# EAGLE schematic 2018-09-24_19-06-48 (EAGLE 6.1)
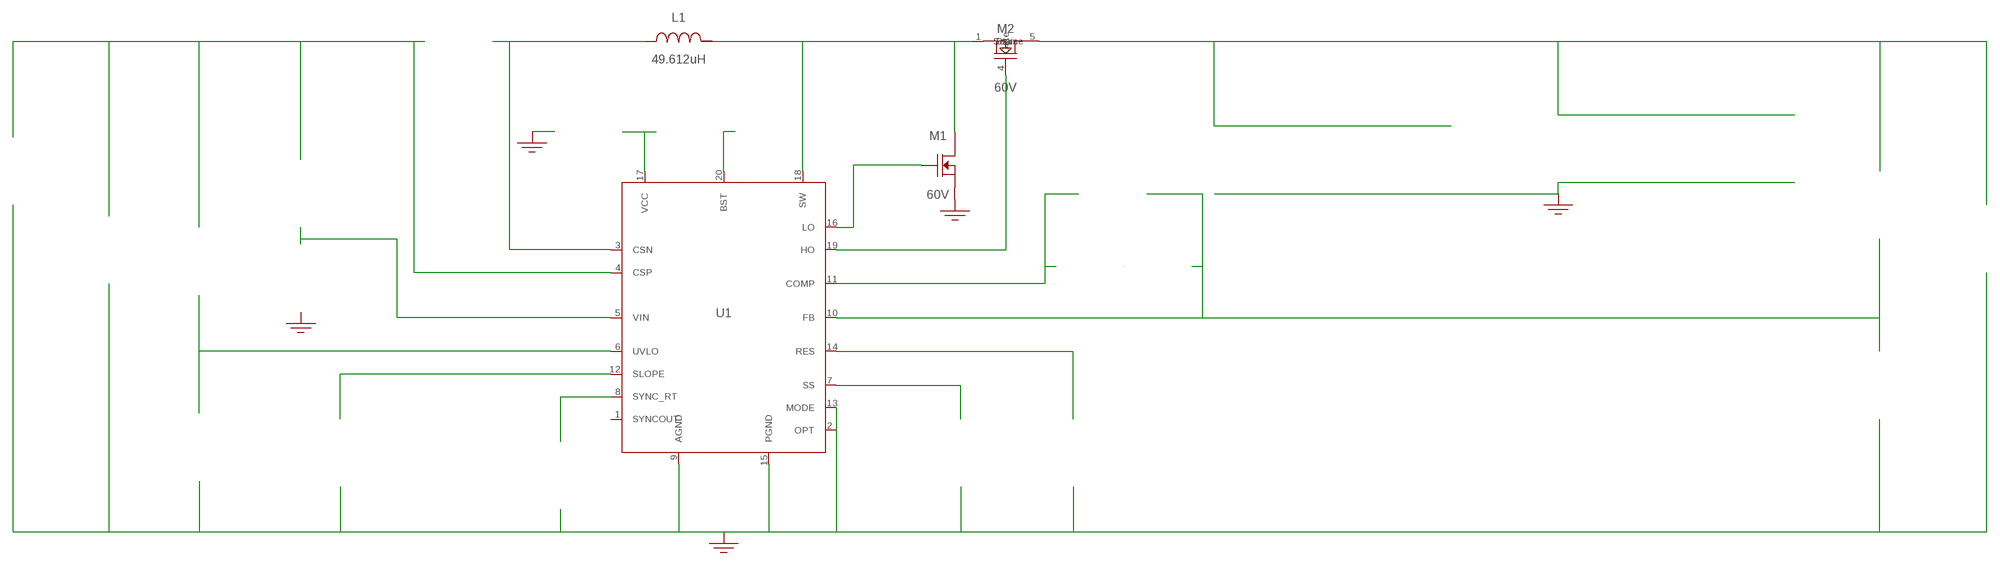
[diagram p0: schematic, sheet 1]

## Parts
CBST  330nF  C1608X5R1H334K080ABC1608X5R1H334K080AB  [0603]  (not placed on a sheet)
CCOMP  27nF  C1812C273J5GACTUC1812C273J5GACTU  [1812]  (not placed on a sheet)
CCOMP2  1.5nF  GCM1885C1H152JA16DGCM1885C1H152JA16D  [0603]  (not placed on a sheet)
CIN  270uF  16SVPG270M16SVPG270M  [CAPSMT_62_C10]  (not placed on a sheet)
COUT  470uF  EEV-FK1J471MEEV-FK1J471M  [SM_RADIAL_J16]  (not placed on a sheet)
COUT_2  470uF  EEV-FK1J471MEEV-FK1J471M  [SM_RADIAL_J16]  (not placed on a sheet)
COUT_3  470uF  EEV-FK1J471MEEV-FK1J471M  [SM_RADIAL_J16]  (not placed on a sheet)
COUT_4  470uF  EEV-FK1J471MEEV-FK1J471M  [SM_RADIAL_J16]  (not placed on a sheet)
COUTX  10uF  CL32B106KBJNNWECL32B106KBJNNWE  [1210_270]  (not placed on a sheet)
COUTX_2  10uF  CL32B106KBJNNWECL32B106KBJNNWE  [1210_270]  (not placed on a sheet)
COUTX_3  10uF  CL32B106KBJNNWECL32B106KBJNNWE  [1210_270]  (not placed on a sheet)
COUTX_4  10uF  CL32B106KBJNNWECL32B106KBJNNWE  [1210_270]  (not placed on a sheet)
CRES  470nF  GRM188R71E474KA12DGRM188R71E474KA12D  [0603]  (not placed on a sheet)
CSS  220nF  GRM155R61A224KE19DGRM155R61A224KE19D  [0402]  (not placed on a sheet)
CVCC  4.7uF  C1608X6S1C475K080ACC1608X6S1C475K080AC  [0603]  (not placed on a sheet)
CVIN  470nF  GRM188R61C474KA93DGRM188R61C474KA93D  [0603]  (not placed on a sheet)
DBST  540mV  XBS104S13R-GXBS104S13R-G  [SOD-323]  (not placed on a sheet)
GND1  WB_GND  WB_GNDWB_GND  [WB_GND]
GND2  WB_GND  WB_GNDWB_GND  [WB_GND]
GND3  WB_GND  WB_GNDWB_GND  [WB_GND]
GND4  WB_GND  WB_GNDWB_GND  [WB_GND]
GND5  WB_GND  WB_GNDWB_GND  [WB_GND]
IOUT  WB_CURRENT_LOAD  WB_CURRENT_LOADWB_CURRENT_LOAD  [WB_CURRENT_LOAD]  (not placed on a sheet)
L1  49.612uH  CUSTOM1CUSTOM1  [GEN_Ind]
M1  60V  CSD18532Q5BCSD18532Q5B  [TRANS_NexFET_Q5B]
M2  60V  CSD18543Q3ACSD18543Q3A  [DNH0008A]
RCOMP  36.5k  RC0201FR-0736K5LRC0201FR-0736K5L  [0201]  (not placed on a sheet)
RFBB  1.6k  RC0603FR-071K6LRC0603FR-071K6L  [0603]  (not placed on a sheet)
RFBT  46.4k  CRCW040246K4FKEDCRCW040246K4FKED  [0402]  (not placed on a sheet)
RSENSE  4m  ERJ-M1WSF4M0UERJ-M1WSF4M0U  [2512]  (not placed on a sheet)
RSLOPE  301k  CRCW0402301KFKEDCRCW0402301KFKED  [0402]  (not placed on a sheet)
RT  162k  RC0201FR-07162KLRC0201FR-07162KL  [0201]  (not placed on a sheet)
RUVB  8.25k  CRCW04028K25FKEDCRCW04028K25FKED  [0402]  (not placed on a sheet)
RUVT  51.1k  CRCW040251K1FKEDCRCW040251K1FKED  [0402]  (not placed on a sheet)
RVIN  2.74  RC1210FR-072R74LRC1210FR-072R74L  [1210]  (not placed on a sheet)
U1  LM5122MH/NOPB  LM5122MH/NOPBLM5122MH/NOPB  [MXA20A]
VIN  WB_BATTERY  WB_BATTERYWB_BATTERY  [WB_BATTERY]  (not placed on a sheet)

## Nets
0: Cin.-@2 Cout.-@2 Cout_2.-@2 Cout_3.-@2 Cout_4.-@2 Coutx.2@2 Coutx_2.2@2 Coutx_3.2@2 Coutx_4.2@2 Cres.2@2 Css.2@2 Cvcc.1@1 Cvin.2@2 GND1.1 GND2.1 GND3.1 GND4.1 GND5.1 Iout.-@2 M1.1(Source) M1.2(Source) M1.3(Source) Rfbb.2@2 Rslope.2@2 Rt.2@2 Ruvb.2@2 U1.2(OPT) U1.9(AGND) U1.13(MODE) U1.15(PGND) U1.21(EP) Vin.-@2
1: Ruvb.1@1 Ruvt.2@2 U1.6(UVLO)
2: Cvin.1@1 Rvin.2@2 U1.5(VIN)
3: Rslope.1@1 U1.12(SLOPE)
4: Cin.+@1 Rsense.1@1 Ruvt.1@1 Rvin.1@1 U1.4(CSP) Vin.+@1
5: L1.1 Rsense.2@2 U1.3(CSN)
6: Rt.1@1 U1.8(SYNC_RT)
7: Cvcc.2@2 Dbst.A@1 U1.17(VCC)
8: Cbst.1@1 Dbst.K@2 U1.20(BST)
9: Css.1@1 U1.7(SS)
10: Cres.1@1 U1.14(RES)
11: Ccomp2.1@1 Ccomp.1@1 Rfbb.1@1 Rfbt.2@2 U1.10(FB)
12: M2.4(Gate) U1.19(HO)
13: M1.4(Gate) U1.16(LO)
14: Ccomp2.2@2 Rcomp.1@1 U1.11(COMP)
15: Cout.+@1 Cout_2.+@1 Cout_3.+@1 Cout_4.+@1 Coutx.1@1 Coutx_2.1@1 Coutx_3.1@1 Coutx_4.1@1 Iout.+@1 M2.5(Drain) M2.6(Drain) M2.7(Drain) M2.8(Drain) M2.9(Drain) Rfbt.1@1
16: Cbst.2@2 L1.2 M1.5(Drain) M1.6(Drain) M1.7(Drain) M1.8(Drain) M1.9(Drain) M2.1(Source) M2.2(Source) M2.3(Source) U1.18(SW)
28: Ccomp.2@2 Rcomp.2@2
Unconnected: CBST.1 CBST.2 CCOMP2.1 CCOMP2.2 CCOMP.1 CCOMP.2 CIN.1(+) CIN.2(-) COUT.1(+) COUT.2(-) COUT_2.1(+) COUT_2.2(-) COUT_3.1(+) COUT_3.2(-) COUT_4.1(+) COUT_4.2(-) COUTX.1 COUTX.2 COUTX_2.1 COUTX_2.2 COUTX_3.1 COUTX_3.2 COUTX_4.1 COUTX_4.2 CRES.1 CRES.2 CSS.1 CSS.2 CVCC.1 CVCC.2 CVIN.1 CVIN.2 DBST.1(K) DBST.2(A) IOUT.1(+) IOUT.2(-) RCOMP.1 RCOMP.2 RFBB.1 RFBB.2 RFBT.1 RFBT.2 RSENSE.1 RSENSE.2 RSLOPE.1 RSLOPE.2 RT.1 RT.2 RUVB.1 RUVB.2 RUVT.1 RUVT.2 RVIN.1 RVIN.2 U1.1(SYNCOUT) VIN.1(+) VIN.2(-)

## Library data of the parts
CBST = AcceleratedDesigns_Lib:C1608X5R1H334K080AB; Cap: 3.3E-7; Datasheet_URL: https://product.tdk.com/en/search/capacitor/ceramic/mlcc/info?part%5Fno%3DC1608X5R1H334K080AB; ESR: 0.016574; IRMS: 1.28367; Manufacturer_Name: TDK; Manufacturer_Part_Number: C1608X5R1H334K080AB; VDC: 50.0; Vendor: TDK
CCOMP = AcceleratedDesigns_Lib:C1812C273J5GACTU; Cap: 2.7E-8; Datasheet_URL: http://www.kemet.com/docfinder?Partnumber%3DC1812C273J5GACTU; ESR: 0.0; IRMS: 0.0; Manufacturer_Name: Kemet; Manufacturer_Part_Number: C1812C273J5GACTU; VDC: 50.0; Vendor: Kemet
CCOMP2 = AcceleratedDesigns_Lib:GCM1885C1H152JA16D; Cap: 1.5E-9; Datasheet_URL: http://www.murata.com/products/catalog/pdf/c03e.pdf; ESR: 0.0; IRMS: 0.0; Manufacturer_Name: MuRata; Manufacturer_Part_Number: GCM1885C1H152JA16D; VDC: 50.0; Vendor: MuRata
CIN = AcceleratedDesigns_Lib:16SVPG270M; Cap: 2.7E-4; Datasheet_URL: %20; ESR: 0.008; IRMS: 5.8; Manufacturer_Name: Panasonic; Manufacturer_Part_Number: 16SVPG270M; VDC: 16.0; Vendor: Panasonic
COUT COUT_2-COUT_4 = AcceleratedDesigns_Lib:EEV-FK1J471M; Cap: 4.7E-4; Datasheet_URL: http://www.panasonic.com/industrial/components/pdf/smt%5Faec%5F050505.pdf; ESR: 0.082; IRMS: 1.41; Manufacturer_Name: Panasonic; Manufacturer_Part_Number: EEV-FK1J471M; VDC: 63.0; Vendor: Panasonic
COUTX COUTX_2-COUTX_4 = AcceleratedDesigns_Lib:CL32B106KBJNNWE; Cap: 1.0E-5; Datasheet_URL: http://www.samsungsem.com/kr/support/product%2Dsearch/mlcc/%5F%5FicsFiles/afieldfile/2016/08/18/S%5FCL32B106KBJNNWE.pdf; ESR: 0.005; IRMS: 0.0; Manufacturer_Name: Samsung Electro-Mechanics; Manufacturer_Part_Number: CL32B106KBJNNWE; VDC: 50.0; Vendor: Samsung Electro-Mechanics
CRES = AcceleratedDesigns_Lib:GRM188R71E474KA12D; Cap: 4.7E-7; ESR: 0.0; IRMS: 0.0; Manufacturer_Name: MuRata; Manufacturer_Part_Number: GRM188R71E474KA12D; VDC: 25.0; Vendor: MuRata
CSS = AcceleratedDesigns_Lib:GRM155R61A224KE19D; Cap: 2.2E-7; ESR: 0.0; IRMS: 0.0; Manufacturer_Name: MuRata; Manufacturer_Part_Number: GRM155R61A224KE19D; VDC: 10.0; Vendor: MuRata
CVCC = AcceleratedDesigns_Lib:C1608X6S1C475K080AC; Cap: 4.7E-6; Datasheet_URL: https://product.tdk.com/en/search/capacitor/ceramic/mlcc/info?part%5Fno%3DC1608X6S1C475K080AC; ESR: 0.003728; IRMS: 2.69359; Manufacturer_Name: TDK; Manufacturer_Part_Number: C1608X6S1C475K080AC; VDC: 16.0; Vendor: TDK
CVIN = AcceleratedDesigns_Lib:GRM188R61C474KA93D; Cap: 4.7E-7; ESR: 0.0; IRMS: 0.0; Manufacturer_Name: MuRata; Manufacturer_Part_Number: GRM188R61C474KA93D; VDC: 16.0; Vendor: MuRata
DBST = AcceleratedDesigns_Lib:XBS104S13R-G; Datasheet_URL: http://www.torexsemi.com/products/schottky%5Fbarrier%5Fdiodes/data/XBS104S13.pdf; Io: 1.0; Manufacturer_Name: Torex USA Corporation; Manufacturer_Part_Number: XBS104S13R-G; VFatIo: 0.54; VRRM: 40.0; Vendor: Torex USA Corporation
GND1-GND5 = AcceleratedDesigns_Lib:WB_GND; Manufacturer_Name: WB_GND; Manufacturer_Part_Number: WB_GND; PowerPortType: POWER_GROUND; Value: Value
IOUT = AcceleratedDesigns_Lib:WB_CURRENT_LOAD; Manufacturer_Name: WB_CURRENT_LOAD; Manufacturer_Part_Number: WB_CURRENT_LOAD; PowerPortType: POWER_GROUND; Value: Value
L1 = AcceleratedDesigns_Lib:CUSTOM1; Budget_Price: 0.0; Component_Type: Inductor; Component_Type_Index: 20; DCR: 0.004592076643867826; Dimension_X: 0.0; Dimension_Y: 0.0; Dimension_Z: 0.0; Foot_Print_Area: 0.0; IDC: 17.815258002748998; IDC_Max: 0.0; L: 4.9612449999311304E-5; Manufacture: CUSTOM; Manufacturer_Name: CUSTOM; Manufacturer_Part_Number: GENERIC_INDUCTOR; Mount: ?; Part_ID: 18; Part_Number: CUSTOM; Quantity: 1; Quantity_In_stock: 0; Schematic_mapping_symbol: WB_INDUCTOR; Technology: ?; Thermal_ID: CUSTOM; Thermal_Status: N; Tolerance: 0.0; Vendor: Unknown
M1 = AcceleratedDesigns_Lib:CSD18532Q5B; Datasheet_URL: http://www.ti.com/lit/ds/symlink/csd18532q5b.pdf; IdsMax: 100.0; Manufacturer_Name: Texas Instruments; Manufacturer_Part_Number: CSD18532Q5B; QgTyp: 21.0; Quantity: 1; Rdson45: 0.0043; VdsMax: 60.0; Vendor: Texas Instruments
M2 = AcceleratedDesigns_Lib:CSD18543Q3A; IdsMax: 20.0; Manufacturer_Name: Texas Instruments; Manufacturer_Part_Number: CSD18543Q3A; QgTyp: 5.3; Quantity: 1; Rdson45: 0.0118; VdsMax: 30.0; Vendor: Texas Instruments
RCOMP = AcceleratedDesigns_Lib:RC0201FR-0736K5L; Datasheet_URL: http://www.yageo.com/documents/recent/PYu%2DRC%5FGroup%5F51%5FRoHS%5FL%5F5.pdf; Manufacturer_Name: Yageo; Manufacturer_Part_Number: RC0201FR-0736K5L; Power: 0.05; Resistance: 36500.0; Tolerance: 1.0; Vendor: Yageo America
RFBB = AcceleratedDesigns_Lib:RC0603FR-071K6L; Manufacturer_Name: Yageo; Manufacturer_Part_Number: RC0603FR-071K6L; Power: 0.1; Resistance: 1600.0; Tolerance: 1.0; Vendor: Yageo America
RFBT = AcceleratedDesigns_Lib:CRCW040246K4FKED; Manufacturer_Name: Vishay-Dale; Manufacturer_Part_Number: CRCW040246K4FKED; Power: 0.063; Resistance: 46400.0; Tolerance: 1.0; Vendor: Vishay-Dale
RSENSE = AcceleratedDesigns_Lib:ERJ-M1WSF4M0U; Manufacturer_Name: Panasonic; Manufacturer_Part_Number: ERJ-M1WSF4M0U; Power: 1.0; Resistance: 0.0040; Tolerance: 1.0; Vendor: Panasonic
RSLOPE = AcceleratedDesigns_Lib:CRCW0402301KFKED; Manufacturer_Name: Vishay-Dale; Manufacturer_Part_Number: CRCW0402301KFKED; Power: 0.063; Resistance: 301000.0; Tolerance: 1.0; Vendor: Vishay-Dale
RT = AcceleratedDesigns_Lib:RC0201FR-07162KL; Datasheet_URL: http://www.yageo.com/documents/recent/PYu%2DRC%5FGroup%5F51%5FRoHS%5FL%5F5.pdf; Manufacturer_Name: Yageo; Manufacturer_Part_Number: RC0201FR-07162KL; Power: 0.05; Resistance: 162000.0; Tolerance: 1.0; Vendor: Yageo America
RUVB = AcceleratedDesigns_Lib:CRCW04028K25FKED; Manufacturer_Name: Vishay-Dale; Manufacturer_Part_Number: CRCW04028K25FKED; Power: 0.063; Resistance: 8250.0; Tolerance: 1.0; Vendor: Vishay-Dale
RUVT = AcceleratedDesigns_Lib:CRCW040251K1FKED; Manufacturer_Name: Vishay-Dale; Manufacturer_Part_Number: CRCW040251K1FKED; Power: 0.063; Resistance: 51100.0; Tolerance: 1.0; Vendor: Vishay-Dale
RVIN = AcceleratedDesigns_Lib:RC1210FR-072R74L; Datasheet_URL: http://www.yageo.com/documents/recent/PYu%2DRC1210%5F51%5FRoHS%5FL%5F%284%29.pdf; Manufacturer_Name: Yageo; Manufacturer_Part_Number: RC1210FR-072R74L; Power: 0.5; Resistance: 2.74; Tolerance: 1.0; Vendor: Yageo
U1 = AcceleratedDesigns_Lib:LM5122MH/NOPB; Datasheet_URL: http://www.ti.com/product/lm5122; Frequency: 1000000.0; Imax: 40.0; Manufacturer_Name: Texas Instruments; Manufacturer_Part_Number: LM5122MH/NOPB; Mktg_Package: MXA20A; NSID: LM5122MH/NOPB; Package: MXA20A; Vendor: Texas Instruments
VIN = AcceleratedDesigns_Lib:WB_BATTERY; Manufacturer_Name: WB_BATTERY; Manufacturer_Part_Number: WB_BATTERY; PowerPortType: POWER_GROUND; Value: Value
